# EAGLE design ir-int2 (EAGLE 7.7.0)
DRAWING_AUTHOR: M. Golicz
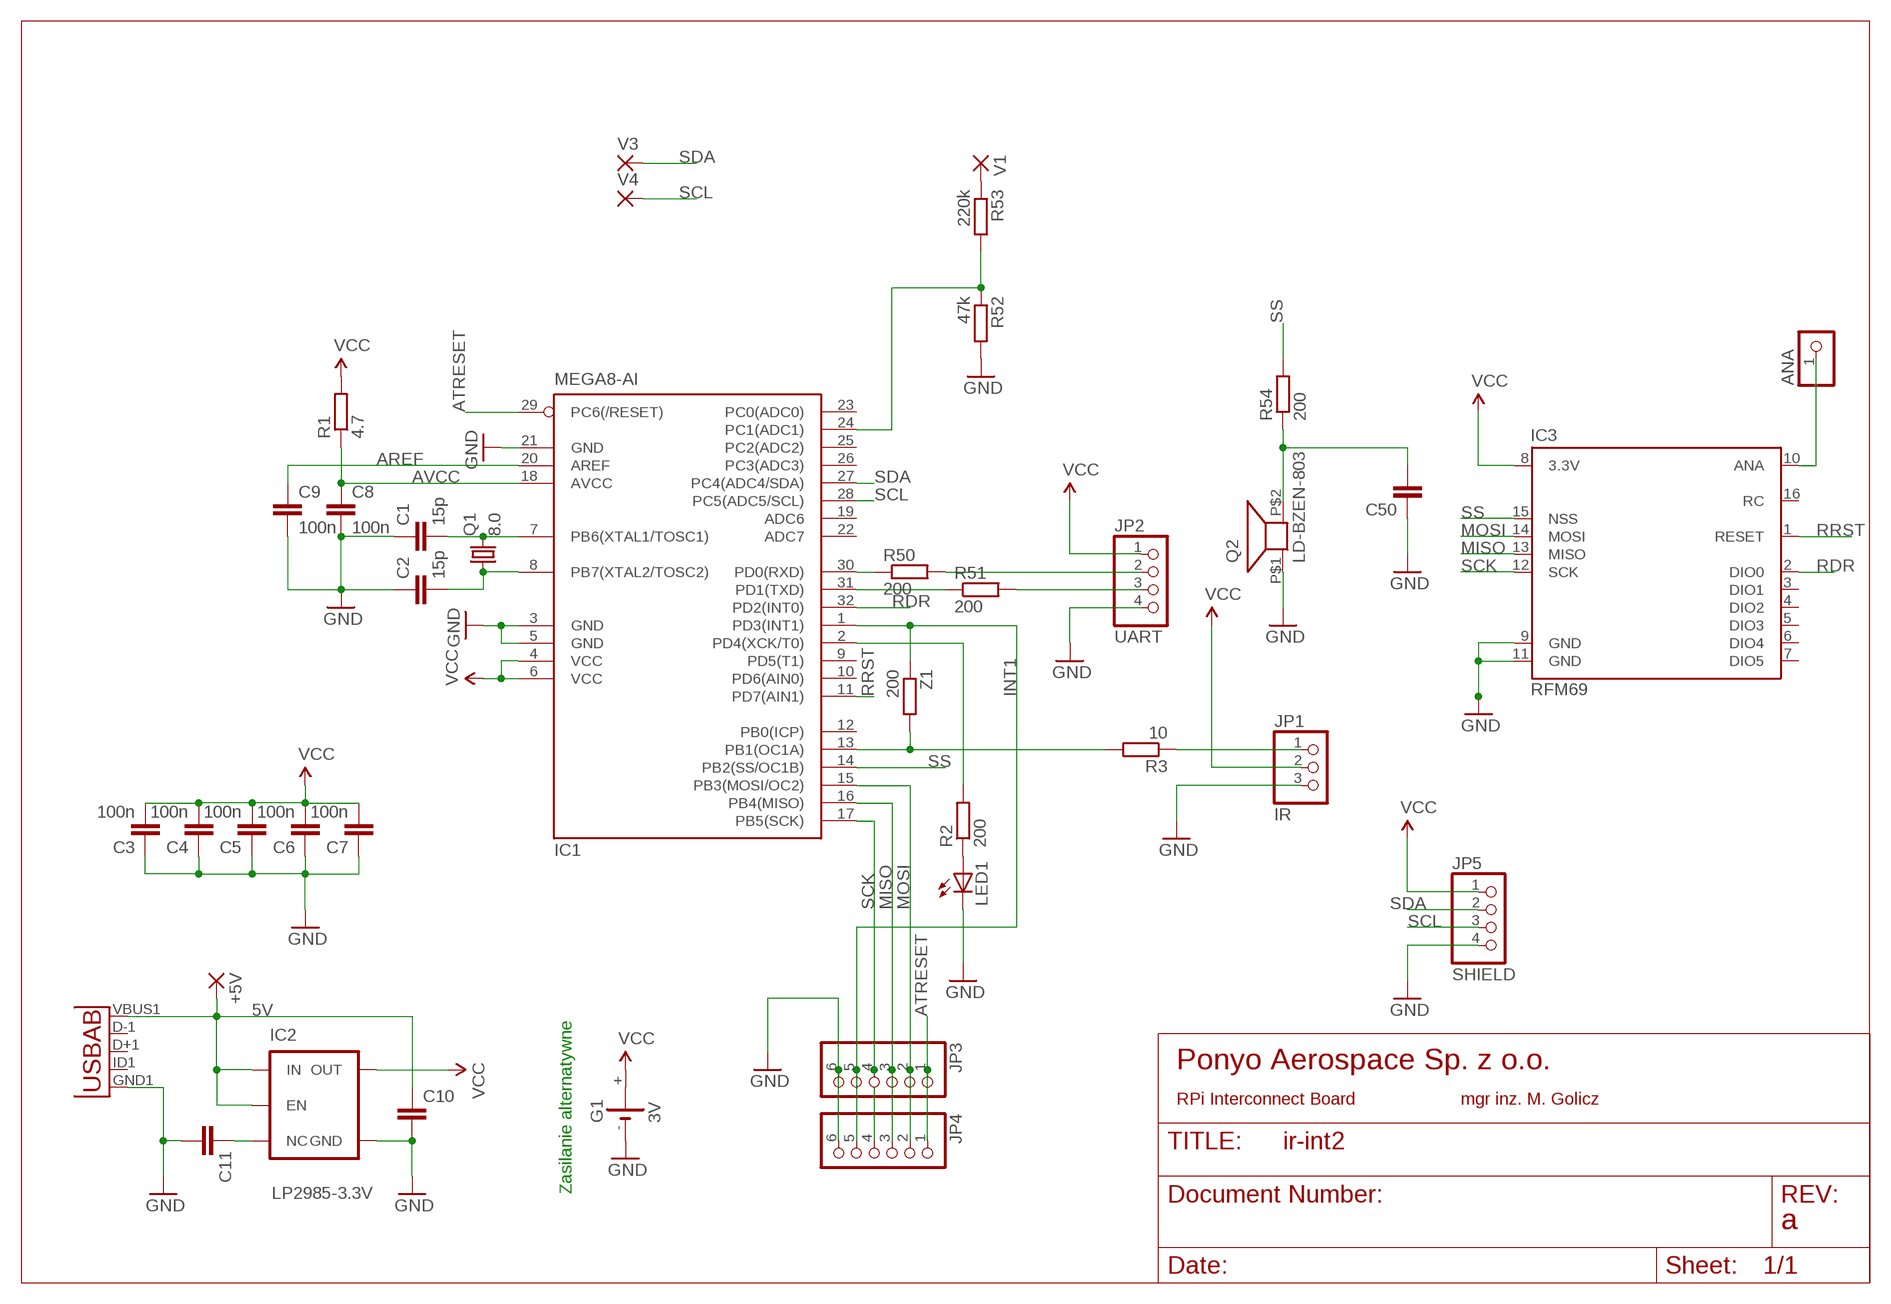
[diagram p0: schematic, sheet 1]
FRAME2 (DINA4_L): PROJECT_NAME: parasite

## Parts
+5V  SMD2  [SMD1,27-2,54]
ANA  PINHD-1X1  [1X01]
C1  15p  C-EUC0805  [C0805]
C2  15p  C-EUC0805  [C0805]
C3  100n  C-EUC0805  [C0805]
C4  100n  C-EUC0805  [C0805]
C5  100n  C-EUC0805  [C0805]
C6  100n  C-EUC0805  [C0805]
C7  100n  C-EUC0805  [C0805]
C8  100n  C-EUC0805  [C0805]
C9  100n  C-EUC0805  [C0805]
C10  C-EUC0805  [C0805]
C11  C-EUC0805  [C0805]
C50  C-EUC0805  [C0805]
G1  3V  CR2032SMD-HOLDER  [CR2032-HOLDER]
IC1  MEGA8-AI  [TQFP32-08]
IC2  LP2985-3.3V  V_REG_TPS76433SOT23-5  [SOT23-5]
IC3  RFM69  [RFM69SMD]
JP1  IR  PINHD-1X3  [1X03]
JP2  UART  PINHD-1X4  [1X04]
JP3  PINHD-1X6  [1X06]
JP4  PINHD-1X6  [1X06]
JP5  SHIELD  PINHD-1X4  [1X04]
LED1  LEDCHIPLED_0805  [CHIPLED_0805]
Q1  8.0  CRYSTALHC49UP  [HC49UP]
Q2  LD-BZEN-803  [BZEN803]
R1  4.7  R-EU_R0805  [R0805]
R2  200  R-EU_R0805  [R0805]
R3  10  R-EU_R0805  [R0805]
R50  200  R-EU_R0805  [R0805]
R51  200  R-EU_R0805  [R0805]
R52  47k  R-EU_R0805  [R0805]
R53  220k  R-EU_R0805  [R0805]
R54  200  R-EU_R0805  [R0805]
U1  USB""  [USB-MICRO-SMD]
V1  SMD2  [SMD1,27-2,54]
V3  SMD2  [SMD1,27-2,54]
V4  SMD2  [SMD1,27-2,54]
Z1  200  R-EU_R0805  [R0805]

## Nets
5V: +5V.1(P) C10.1 IC2.1(IN) IC2.3(EN) U1.VBUS1(VBUS)
ADC: IC1.24(PC1(ADC1)) R52.1 R53.2
ANA: ANA.1 IC3.10(ANA)
AREF: C9.1 IC1.20(AREF)
ATRESET: IC1.29(PC6(/RESET)) JP3.1 JP4.1
AVCC: C8.1 IC1.18(AVCC) R1.1
GND: C1.1 C2.1 C3.1 C4.1 C5.1 C6.1 C7.1 C8.2 C9.2 C10.2 C11.2 C50.1 G1.- IC1.3(GND) IC1.5(GND) IC1.21(GND) IC2.2(GND) IC3.9(GND) IC3.11(GND) JP1.3 JP2.4 JP3.6 JP4.6 JP5.4 LED1.C Q2.P$1 R52.2 U1.GND1(GND)
INT1: IC1.1(PD3(INT1)) JP3.5 JP4.5 Z1.1
IR: IC1.13(PB1(OC1A)) R3.2 Z1.2
LED: IC1.2(PD4(XCK/T0)) R2.2
MISO: IC1.16(PB4(MISO)) IC3.13(MISO) JP3.3 JP4.3
MOSI: IC1.15(PB3(MOSI/OC2)) IC3.14(MOSI) JP3.2 JP4.2
N$1: JP1.1 R3.1
N$2: C50.2 Q2.P$2 R54.1
N$3: JP2.2 R50.2
N$4: JP2.3 R51.2
N$5: C11.1 IC2.4(NC)
N$6: JP4.4
N$7: R53.1 V1.1(P)
N$29: LED1.A R2.1
Q1: C1.2 IC1.7(PB6(XTAL1/TOSC1)) Q1.2
Q2: C2.2 IC1.8(PB7(XTAL2/TOSC2)) Q1.1
RDR: IC1.32(PD2(INT0)) IC3.2(DIO0)
RRST: IC1.11(PD7(AIN1)) IC3.1(RESET)
RXD: IC1.30(PD0(RXD)) R50.1
SCK: IC1.17(PB5(SCK)) IC3.12(SCK) JP3.4
SCL: IC1.28(PC5(ADC5/SCL)) JP5.3 V4.1(P)
SDA: IC1.27(PC4(ADC4/SDA)) JP5.2 V3.1(P)
SS: IC1.14(PB2(SS/OC1B)) IC3.15(NSS) R54.2
TXD: IC1.31(PD1(TXD)) R51.1
VCC: C3.2 C4.2 C5.2 C6.2 C7.2 G1.+ IC1.4(VCC) IC1.6(VCC) IC2.5(OUT) IC3.8(3.3V) JP1.2 JP2.1 JP5.1 R1.2
Unconnected: IC1.9(PD5(T1)) IC1.10(PD6(AIN0)) IC1.12(PB0(ICP)) IC1.19(ADC6) IC1.22(ADC7) IC1.23(PC0(ADC0)) IC1.25(PC2(ADC2)) IC1.26(PC3(ADC3)) IC3.3(DIO1) IC3.4(DIO2) IC3.5(DIO3) IC3.6(DIO4) IC3.7(DIO5) U1.D+1(D+) U1.D-1(D-) U1.ID1(USBID)

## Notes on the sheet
- Ponyo Aerospace Sp. z o.o.
- RPi Interconnect Board | mgr inz. M. Golicz
- Zasilanie alternatywne
- a

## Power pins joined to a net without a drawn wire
RC: IC3.16(RC)

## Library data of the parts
+5V V1 V3 V4 = wirepad:SMD2: SMD PAD
ANA = pinhead:PINHD-1X1: PIN HEADER
C1-C11 C50 = rcl:C-EU: CAPACITOR, European symbol
G1 = XYKlib:CR2032: CR2032 BATTERY CR2032 20MM Coin Cell Battery Holders
IC1 = atmel:MEGA8: MICROCONTROLLER 8 Kbytes FLASH, 1 kbytes SRAM, 512 bytes EEPROM, USART, 6-channel 10 bit ADC, 2-channel 8 bit ADC Pin compatible with Atmega48, ATMega88, ATMega168 Source: avr.lbr; MPN: ATMEGA8-16AU; OC_FARNELL: 9171371; OC_NEWARK: 73M8863
IC2 = SparkFun:V_REG_TPS76433: Voltage Regulator Older TI part. LDO 150mA regulator. No output by-pass cap option. See V_REG_LDO for a better part.
IC3 = SWP:RFM69
JP1 = pinhead:PINHD-1X3: PIN HEADER
JP2 JP5 = pinhead:PINHD-1X4: PIN HEADER
JP3 JP4 = pinhead:PINHD-1X6: PIN HEADER
LED1 = led:LED: LED
Q1 = crystal:CRYSTAL: CRYSTAL; OC_FARNELL: unknown; OC_NEWARK: unknown
Q2 = moi:LD-BZEN-803
R1-R3 R50-R54 Z1 = rcl:R-EU_: RESISTOR, European symbol
U1 = MicroUSB:USB: This is a USB AB connector that is compatible with USB OTG. i.e. this connector can serve as a host or device

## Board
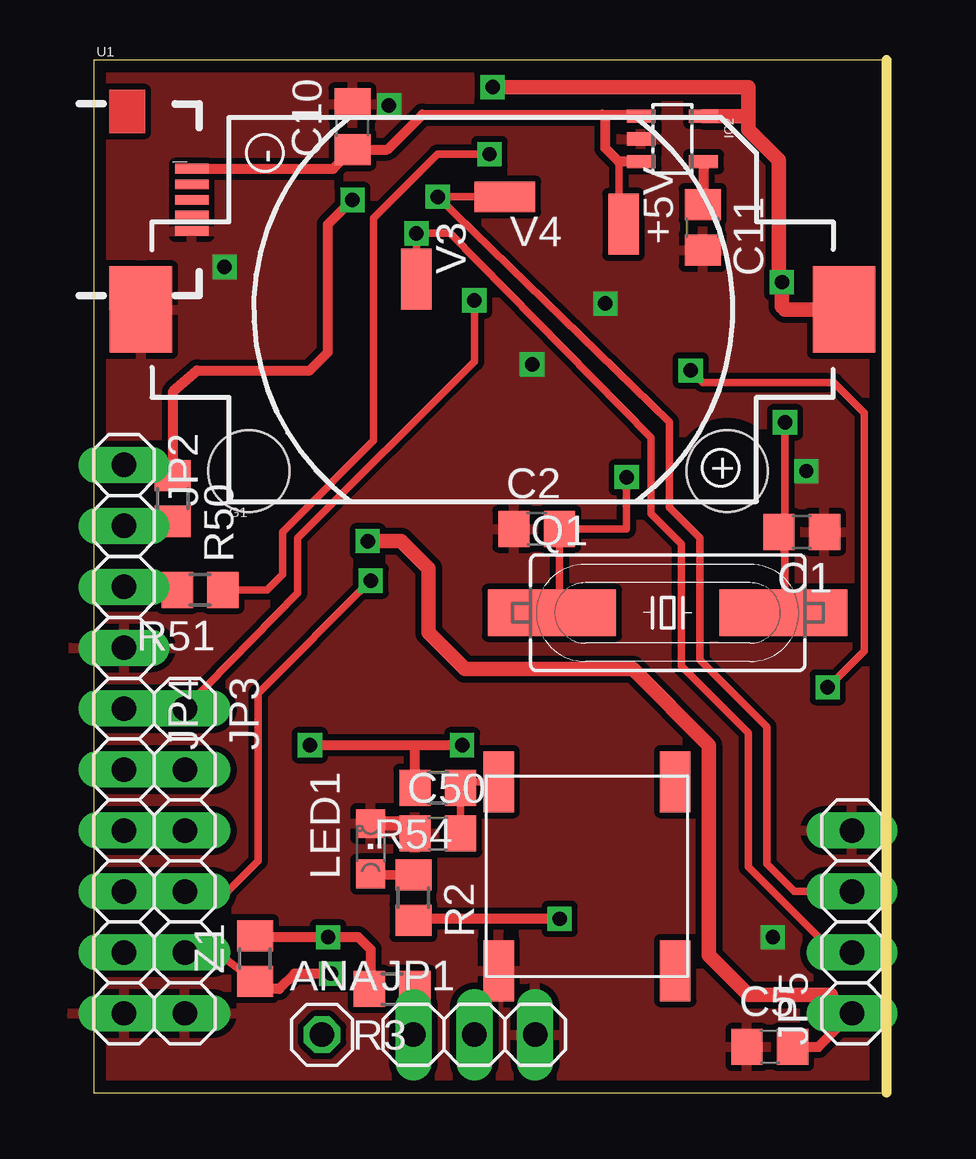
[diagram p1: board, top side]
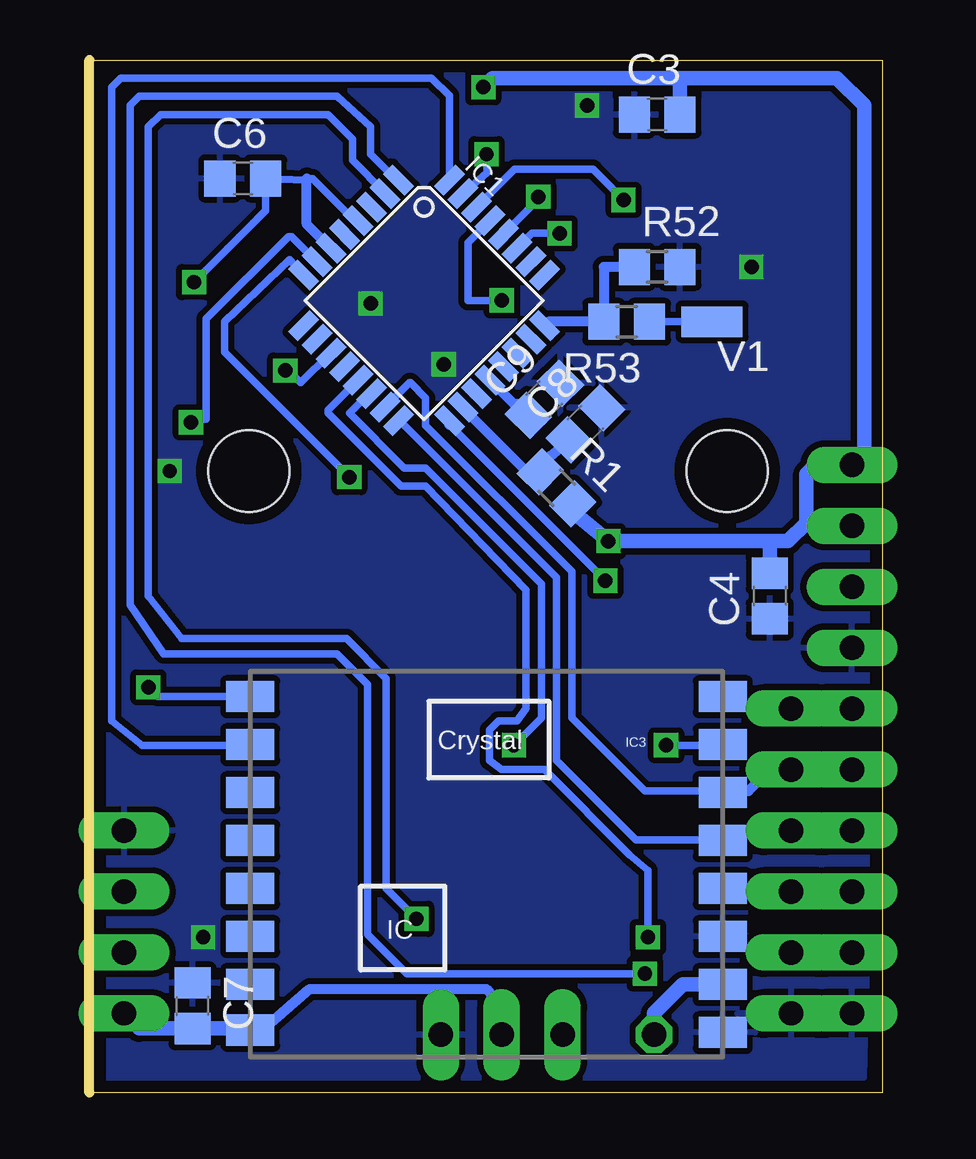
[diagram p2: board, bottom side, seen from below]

Size 33.07 x 43.04 mm. Coordinates in mm from the lower left corner, seen from the top.
Outline: 0,0 33.07,0 33.07,43.04 0,43.04 0,0
Copper layers (1*16): Top 0.035mm / dielectric 1.5mm / Bottom 0.035mm
Design rules "default *": minimum track width 10mil, minimum drill 24mil, track to track 10mil, track to pad 10mil, pad to pad 10mil, via to via 10mil, smd to smd 8mil, copper to edge 20mil, drill to drill 8mil, minimum pad ring 10mil, minimum via ring 8mil, stop-mask expansion 4mil, vias tented up to drill 0mil, thermal gap 10mil
Holes 3.4 mm at 6.48,25.91 26.42,25.91

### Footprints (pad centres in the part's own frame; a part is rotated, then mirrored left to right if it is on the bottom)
SMD1,27-2,54 = smd 1.27 x 2.54: 1 0,0
1X01 = drill 1.016 octagon: 1 0,0
C0805 = smd 1.3 x 1.5: 1 -0.95,0; 2 0.95,0
CR2032-HOLDER = smd 2.591 x 3.607: + 14.656,0; - -14.656,0
TQFP32-08 = smd 1.27 x 0.559: 1 -4.293,2.8; 2 -4.293,2; 3 -4.293,1.2; 4 -4.293,0.4; 5 -4.293,-0.4; 6 -4.293,-1.2; 7 -4.293,-2; 8 -4.293,-2.8; 17 4.293,-2.8; 18 4.293,-2; 19 4.293,-1.2; 20 4.293,-0.4; 21 4.293,0.4; 22 4.293,1.2; 23 4.293,2; 24 4.293,2.8 | smd 0.559 x 1.27: 9 -2.8,-4.293; 10 -2,-4.293; 11 -1.2,-4.293; 12 -0.4,-4.293; 13 0.4,-4.293; 14 1.2,-4.293; 15 2,-4.293; 16 2.8,-4.293; 25 2.8,4.293; 26 2,4.293; 27 1.2,4.293; 28 0.4,4.293; 29 -0.4,4.293; 30 -1.2,4.293; 31 -2,4.293; 32 -2.8,4.293
SOT23-5 = smd 0.55 x 1.2: 1 -0.95,-1.3; 2 0,-1.3; 3 0.95,-1.3; 4 0.95,1.3; 5 -0.95,1.3
RFM69SMD = smd 2 x 1.3: 1 -10.1,6.6; 2 -10.1,4.6; 3 -10.1,2.6; 4 -10.1,0.6; 5 -10.1,-1.4; 6 -10.1,-3.4; 7 -10.1,-5.4; 8 -10.1,-7.3; 9 9.6,-7.4; 10 9.6,-5.4; 11 9.6,-3.4; 12 9.6,-1.4; 13 9.6,0.6; 14 9.6,2.6; 15 9.6,4.6; 16 9.6,6.6
1X03 = drill 1.016 long: 1 -2.54,0; 2 0,0; 3 2.54,0
1X04 = drill 1.016 long: 1 -3.81,0; 2 -1.27,0; 3 1.27,0; 4 3.81,0
1X06 = drill 1.016 long: 1 -6.35,0; 2 -3.81,0; 3 -1.27,0; 4 1.27,0; 5 3.81,0; 6 6.35,0
CHIPLED_0805 = smd 1.2 x 1.2: A 0,-1.05; C 0,1.05
HC49UP = smd 5.334 x 1.93: 1 -4.826,0; 2 4.826,0
BZEN803 = smd 2.54 x 1.27: P$1 -4.064,3.556; P$2 3.81,3.556; P$3 3.81,-3.81; P$4 -4.064,-3.81
R0805 = smd 1.3 x 1.5: 1 -0.95,0; 2 0.95,0
USB-MICRO-SMD = smd 1.4 x 0.4: D+1 2.7,0; D-1 2.7,0.65; GND1 2.7,-1.3; ID1 2.7,-0.65; VBUS1 2.7,1.3

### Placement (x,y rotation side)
+5V  22.1,36.2 180 top
ANA  9.53,2.41 0 top
C1  29.53,23.37 180 top
C2  18.48,23.5 0 top
C3  9.4,40.77 0 bottom
C4  4.7,20.7 90 bottom
C5  28.19,1.91 0 top
C6  26.67,38.1 0 bottom
C7  28.77,3.62 270 bottom
C8  12.38,27.88 45 bottom
C9  14.1,28.89 45 bottom
C10  10.79,40.26 90 top
C11  25.4,36.07 270 top
C50  14.35,10.79 0 top
G1  16.64,32.64 0 top
IC1  19.11,33.02 315 bottom
IC2  24.13,39.75 270 top
IC3  16.26,9.91 0 bottom
JP1  15.88,2.41 0 top
JP2  1.27,22.35 270 top
JP3  3.81,9.65 270 top
JP4  1.27,9.65 270 top
JP5  31.62,7.11 90 top
LED1  11.56,10.16 0 top
Q1  23.94,20 0 top
Q2  20.45,9.14 90 top
R1  13.59,25.21 315 bottom
R2  13.34,8.13 270 top
R3  12.45,4.32 180 top
R50  3.3,24.77 270 top
R51  4.45,20.95 180 top
R52  9.4,34.42 0 bottom
R53  10.67,32.13 180 bottom
R54  14.35,12.7 180 top
U1  1.4,37.21 0 top
V1  7.11,32.13 90 bottom
V3  13.46,33.91 180 top
V4  17.14,37.34 90 top
Z1  6.73,5.59 90 top

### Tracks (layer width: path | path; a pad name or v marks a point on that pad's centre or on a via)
5V
  Top 0.305: 22.76,40.77 IC2.1 | 21.34,40.64 21.21,40.77 | 21.91,38.8 21.91,36.39 +5V.1
  Top 0.406: 22.76,40.77 21.21,40.77 13.72,40.77 12.26,39.31 C10.1 10,38.51 U1.VBUS1 | IC2.3 21.91,38.8 21.34,39.37 21.34,40.64
ADC
  Bottom 0.305: 13.93,32.13 IC1.24
  Bottom 0.406: 13.93,32.13 R53.2 11.62,34.42 R52.1
ANA
  Bottom 0.61: IC3.10 8.32,4.51 9.53,3.3 ANA.1
AREF
  Bottom 0.406: IC1.20 15.37,28.7 15.25,28.7 C9.1
ATRESET  (via drill 0.6)
  Top 0.305: JP3.1 8.51,20.83 8.51,23.11 15.88,30.48 v15.88,33.02
  Top 0.406: JP3.1 JP4.1
  Bottom 0.254: IC1.29 16.36,36.47 16.23,36.47
  Bottom 0.305: IC1.29 17.27,35.43 17.27,33.02 v15.88,33.02
  Bottom 0.406: IC1.29
AVCC
  Bottom 0.305: 13.84,26.54 13.84,26.3 R1.1
  Bottom 0.406: 13.84,26.54 C8.1 | IC1.18 17.49,28.54 14.86,25.91 14.29,25.91 R1.1
GND  (via drill 0.6)
  Top 0.61: LED1.C 12.99,11.21 C50.1
  Bottom 0.406: IC1.21
  other vias: 21.34,32.89 28.32,6.48 29.72,25.91 12.32,41.15 18.29,30.35 5.46,34.42
  pour Top: -0.76,43.69 33.91,43.56 33.78,-0.51 -0.89,-0.38
  pour Bottom: -1.27,74.42 37.34,74.42 39.24,0.64 0.76,0.64 -1.14,74.04 -1.14,74.3
INT1  (via drill 0.6)
  Top 0.305: 6.8,4.32 Z1.1 5.14,5.84 JP3.5
  Top 0.406: JP4.5 JP3.5 | v9.91,4.95 8.38,4.95 7.75,4.32 6.8,4.32
  Bottom 0.305: IC1.1 20.25,38.03 21.34,39.12 21.34,40.26 22.73,41.53 30.99,41.53 31.37,41.15 31.37,20.32 29.97,18.29 22.73,18.29 21.46,17.02 21.46,6.6 19.81,4.95 v9.91,4.95
IR  (via drill 0.6)
  Top 0.305: 7.05,6.22 Z1.2 6.79,6.48 | 11.56,4.38 R3.2
  Top 0.406: 11.56,4.38 11.56,5.97 11.05,6.48 v9.78,6.48 6.79,6.48
  Bottom 0.305: IC1.13 23.11,28.45 23.11,28.32 20.07,25.27 19.05,25.27 14.86,20.95 14.86,16 15.24,15.49 16,15.49 16.38,15.11 16.38,13.84 15.88,13.46 14.1,13.46 10.54,9.91 9.78,9.27 v9.78,6.48
LED  (via drill 0.6)
  Top 0.305: 13.4,7.24 R2.2
  Top 0.406: v19.43,7.24 13.4,7.24
  Bottom 0.305: IC1.2 20.73,37.5 22.1,38.86 22.1,39.75 23.11,40.77 30.1,40.77 30.61,40.26 30.61,20.7 29.21,18.92 22.35,18.92 20.7,17.27 20.7,8.51 v19.43,7.24
MISO
  Top 0.406: JP4.3 JP3.3
  Bottom 0.305: IC1.16 20.13,28 13.59,21.46 13.59,13.84 10.29,10.54 6.69,10.54 IC3.13
  Bottom 0.406: JP3.3 6.24,10.92 IC3.13
MOSI
  Top 0.406: JP4.2 JP3.2
  Bottom 0.305: 6.59,12.57 9.91,12.57 12.95,15.62 12.95,21.72 19.05,27.81 19.05,28.96 19.68,29.59 19.71,29.59 IC1.15
  Bottom 0.406: JP3.2 4.7,13.46 5.59,12.57 6.59,12.57 IC3.14
N$1
  Top 0.406: R3.1 13.4,2.47 JP1.1
N$2
  Top 0.305: Q2.P$2 15.55,12.95 R54.1 C50.2
N$3
  Top 0.305: 3.62,23.62 R50.2
  Top 0.406: JP2.2 3.62,23.62
N$4
  Top 0.305: 1.4,20.95 JP2.3
  Top 0.406: R51.2 1.4,20.95
N$5
  Top 0.406: IC2.4 25.43,37.05 C11.1
N$7
  Bottom 0.305: V1.1 R53.1
N$29
  Top 0.305: 13.31,9.05 R2.1
  Top 0.406: LED1.A 13.31,9.05
Q1  (via drill 0.6)
  Top 0.305: v28.83,27.94 28.83,22.48 | 28.83,22.48 C1.2 | 28.83,22.48 28.83,20.07 Q1.2
  Bottom 0.305: IC1.7 23.59,34.64 24.64,35.69 24.77,35.69 28.19,32.26 28.19,28.07 v28.83,27.94
Q2  (via drill 0.6)
  Top 0.305: v22.23,25.65 22.23,23.5 C2.2 19.43,20.32 Q1.1
  Bottom 0.305: IC1.8 24.73,34.71 27.43,32.13 27.43,30.86 v22.23,25.65
RDR
  Bottom 0.305: IC1.32 18.06,41.55 18.8,42.29 31.75,42.29 32.13,41.91 32.13,15.49 30.86,14.48 26.38,14.48 IC3.2
RRST  (via drill 0.6)
  Top 0.305: v30.61,16.89 32.13,18.41 32.13,28.32 30.86,29.59 25.4,29.59 v24.89,30.1
  Bottom 0.305: IC3.1 30.22,16.51 v30.61,16.89 | v24.89,30.1 24.77,30.1 24.26,29.59 23.02,30.83 IC1.11
RXD  (via drill 0.6)
  Top 0.406: v10.79,37.21 9.78,36.2 9.78,30.86 9.02,30.1 4.32,30.1 3.3,29.21 R50.1
  Bottom 0.305: v10.79,37.21 12.06,38.48 15.35,38.48 IC1.30
SCK  (via drill 0.6)
  Top 0.305: v11.56,21.34 6.86,16.64 6.86,9.65 5.59,8.38 JP3.4
  Bottom 0.305: 18.06,27.84 v11.56,21.34
  Bottom 0.406: JP3.4 6.53,8.38 IC3.12 | IC1.17 18.06,27.84
SCL  (via drill 0.6)
  Top 0.305: JP5.3 29.21,8.38 28.07,9.53 28.07,15.24 25.27,18.03 25.27,23.11 24,24.38 24,27.94 v14.35,37.34 V4.1
  Bottom 0.305: v14.35,37.34 14.36,37.21 IC1.28
SDA  (via drill 0.6)
  Top 0.305: JP5.2 30.86,5.84 27.3,9.4 27.3,14.99 24.51,17.78 24.51,22.86 23.24,24.13 23.24,27.3 14.86,35.81 v13.46,35.81 V3.1
  Bottom 0.305: v13.46,35.81 14.62,35.81 IC1.27
SS  (via drill 0.6)
  Top 0.305: 13.4,14.42 13.46,14.48
  Top 0.406: v15.37,14.48 13.46,14.48 v9.02,14.48 | R54.2 13.4,14.42
  Bottom 0.305: IC1.14 21.41,29.14 22.23,28.32 19.94,26.04 19.05,26.04 14.22,21.21 14.22,15.62 v15.37,14.48 | v9.02,14.48 6.68,14.48 IC3.15
TXD  (via drill 0.6)
  Top 0.305: v16.51,39.12 14.35,39.12 11.68,36.45 11.68,27.18 7.87,23.37 7.87,21.59 7.24,20.95 R51.1
  Bottom 0.254: IC1.31 17.49,37.63
  Bottom 0.305: v16.51,39.12 16.48,38.35 IC1.31
VCC  (via drill 0.6)
  Top 0.305: 28.57,33.91 v28.7,33.78
  Top 0.406: 30.73,4.06 JP5.1 30.23,1.91 C5.2 | 28.7,32.77 28.83,32.64 | 27.24,40.7 27.3,40.77
  Top 0.61: G1.+ 28.83,32.64 | 30.73,4.06 27.3,4.06 25.65,5.71 25.65,14.48 22.48,17.65 15.49,17.65 13.97,19.18 13.97,21.84 12.83,22.99 v11.43,22.99 | v28.7,33.78 28.7,32.77 | v16.64,41.91 27.3,41.91 27.3,40.77 27.3,40.13 28.57,38.86 28.57,33.91 | IC2.5 27.24,40.7
  Bottom 0.305: 21.93,36.34 22.44,36.79 23.75,38.1 24,38.1 | 24,38.1 | 24,38.03 C6.2 25.72,36.76 v28.7,33.78 | 26.42,2.67 IC3.8 25.84,2.61 | 12.92,24.22 R1.2 12.8,24.54
  Bottom 0.406: IC1.6 23.02,35.21 24,36.2 24,38.03 24,38.1 | IC1.4 21.93,36.34 | 30.99,2.67 JP5.1 | 25.84,2.61 23.88,4.32 16.51,4.32 15.88,3.56 JP1.2 | 1.4,26.04 JP2.1 | 4.7,22.86 4.83,22.99 | 8.45,42.1 8.64,42.29
  Bottom 0.61: 30.99,2.67 C7.2 26.42,2.67 | 12.92,24.22 v11.43,22.99 4.83,22.99 3.94,22.99 3.17,23.75 3.17,25.78 2.92,26.04 1.4,26.04 | v16.64,41.91 16.26,42.29 8.64,42.29 1.91,42.29 0.76,41.15 0.76,26.67 JP2.1 | C4.2 4.7,22.86 | C3.2 8.45,42.1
